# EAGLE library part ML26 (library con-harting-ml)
HARTING
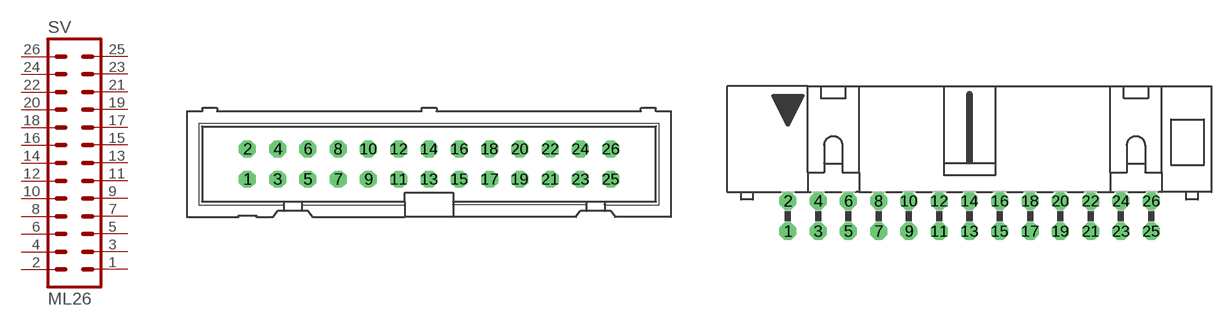
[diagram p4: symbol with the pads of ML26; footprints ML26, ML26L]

Designator prefix SV

## ML26 (OC_FARNELL: unknown; OC_NEWARK: unknown)  [ML26]
1  1  pas
2  2  pas
3  3  pas
4  4  pas
5  5  pas
6  6  pas
7  7  pas
8  8  pas
9  9  pas
10  10  pas
11  11  pas
12  12  pas
13  13  pas
14  14  pas
15  15  pas
16  16  pas
17  17  pas
18  18  pas
19  19  pas
20  20  pas
21  21  pas
22  22  pas
23  23  pas
24  24  pas
25  25  pas
26  26  pas

## ML26L (OC_FARNELL: unknown; OC_NEWARK: unknown)  [ML26L]
Pads as for ML26

## ML263M (OC_FARNELL: unknown; OC_NEWARK: unknown)  [3M_26]
Pads as for ML26

## ML263ML (OC_FARNELL: unknown; OC_NEWARK: unknown)  [3M_26L]
Pads as for ML26

## Footprint ML26 (pad centres in mm)
HARTING
drill 0.914 octagon: 1 -15.24,-1.27; 2 -15.24,1.27; 3 -12.7,-1.27; 4 -12.7,1.27; 5 -10.16,-1.27; 6 -10.16,1.27; 7 -7.62,-1.27; 8 -7.62,1.27; 9 -5.08,-1.27; 10 -5.08,1.27; 11 -2.54,-1.27; 12 -2.54,1.27; 13 0,-1.27; 14 0,1.27; 15 2.54,-1.27; 16 2.54,1.27; 17 5.08,-1.27; 18 5.08,1.27; 19 7.62,-1.27; 20 7.62,1.27; 21 10.16,-1.27; 22 10.16,1.27; 23 12.7,-1.27; 24 12.7,1.27; 25 15.24,-1.27; 26 15.24,1.27

## Footprint ML26L (pad centres in mm)
HARTING
drill 0.914 octagon: 1 -15.24,-1.27; 2 -15.24,1.27; 3 -12.7,-1.27; 4 -12.7,1.27; 5 -10.16,-1.27; 6 -10.16,1.27; 7 -7.62,-1.27; 8 -7.62,1.27; 9 -5.08,-1.27; 10 -5.08,1.27; 11 -2.54,-1.27; 12 -2.54,1.27; 13 0,-1.27; 14 0,1.27; 15 2.54,-1.27; 16 2.54,1.27; 17 5.08,-1.27; 18 5.08,1.27; 19 7.62,-1.27; 20 7.62,1.27; 21 10.16,-1.27; 22 10.16,1.27; 23 12.7,-1.27; 24 12.7,1.27; 25 15.24,-1.27; 26 15.24,1.27

## Footprint 3M_26 (pad centres in mm)
3M
drill 0.813 square: 1 -15.24,-1.27; 2 -15.24,1.27; 3 -12.7,-1.27; 4 -12.7,1.27; 5 -10.16,-1.27; 6 -10.16,1.27; 7 -7.62,-1.27; 8 -7.62,1.27; 9 -5.08,-1.27; 10 -5.08,1.27; 11 -2.54,-1.27; 12 -2.54,1.27; 13 0,-1.27; 14 0,1.27; 15 2.54,-1.27; 16 2.54,1.27; 17 5.08,-1.27; 18 5.08,1.27; 19 7.62,-1.27; 20 7.62,1.27; 21 10.16,-1.27; 22 10.16,1.27; 23 12.7,-1.27; 24 12.7,1.27; 25 15.24,-1.27; 26 15.24,1.27

## Footprint 3M_26L (pad centres in mm)
3M
drill 0.813 square: 1 -15.24,-5.08; 2 -15.24,-2.54; 3 -12.7,-5.08; 4 -12.7,-2.54; 5 -10.16,-5.08; 6 -10.16,-2.54; 7 -7.62,-5.08; 8 -7.62,-2.54; 9 -5.08,-5.08; 10 -5.08,-2.54; 11 -2.54,-5.08; 12 -2.54,-2.54; 13 0,-5.08; 14 0,-2.54; 15 2.54,-5.08; 16 2.54,-2.54; 17 5.08,-5.08; 18 5.08,-2.54; 19 7.62,-5.08; 20 7.62,-2.54; 21 10.16,-5.08; 22 10.16,-2.54; 23 12.7,-5.08; 24 12.7,-2.54; 25 15.24,-5.08; 26 15.24,-2.54
hole 2.54 at -21.158,-3.277
hole 2.54 at 21.158,-3.277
